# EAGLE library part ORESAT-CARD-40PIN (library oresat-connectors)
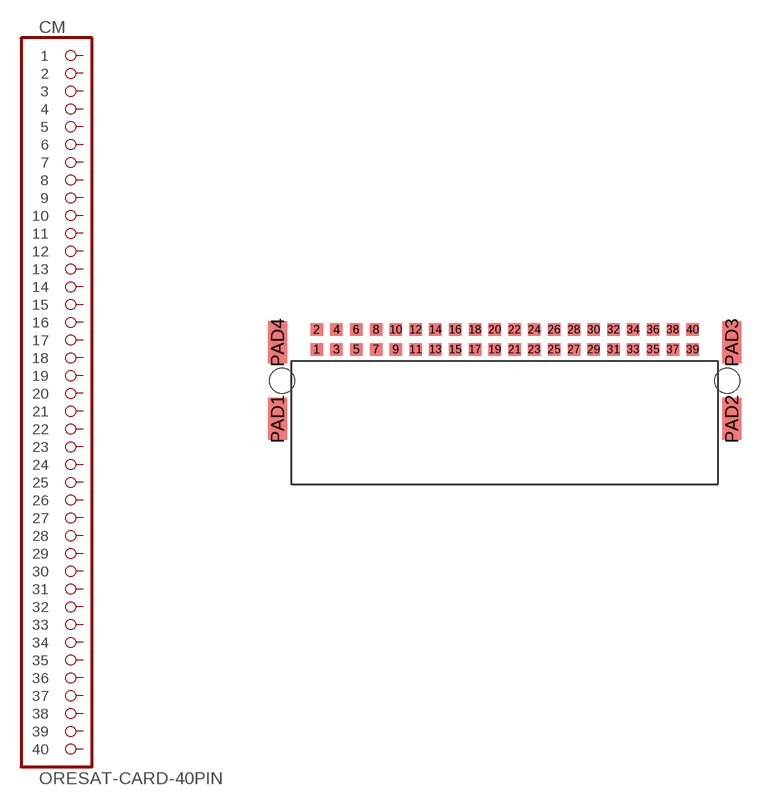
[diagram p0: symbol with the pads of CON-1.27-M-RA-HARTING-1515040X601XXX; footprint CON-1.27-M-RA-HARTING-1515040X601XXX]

Designator prefix CM

## ORESAT-CARD-40PIN  [CON-1.27-M-RA-HARTING-1515040X601XXX]
1  1  pas
2  2  pas
3  3  pas
4  4  pas
5  5  pas
6  6  pas
7  7  pas
8  8  pas
9  9  pas
10  10  pas
11  11  pas
12  12  pas
13  13  pas
14  14  pas
15  15  pas
16  16  pas
17  17  pas
18  18  pas
19  19  pas
20  20  pas
21  21  pas
22  22  pas
23  23  pas
24  24  pas
25  25  pas
26  26  pas
27  27  pas
28  28  pas
29  29  pas
30  30  pas
31  31  pas
32  32  pas
33  33  pas
34  34  pas
35  35  pas
36  36  pas
37  37  pas
38  38  pas
39  39  pas
40  40  pas

## Footprint CON-1.27-M-RA-HARTING-1515040X601XXX (pad centres in mm)
smd 0.8 x 0.8: 1 -12.065,2; 2 -12.065,3.27; 3 -10.795,2; 4 -10.795,3.27; 5 -9.525,2; 6 -9.525,3.27; 7 -8.255,2; 8 -8.255,3.27; 9 -6.985,2; 10 -6.985,3.27; 11 -5.715,2; 12 -5.715,3.27; 13 -4.445,2; 14 -4.445,3.27; 15 -3.175,2; 16 -3.175,3.27; 17 -1.905,2; 18 -1.905,3.27; 19 -0.635,2; 20 -0.635,3.27; 21 0.635,2; 22 0.635,3.27; 23 1.905,2; 24 1.905,3.27; 25 3.175,2; 26 3.175,3.27; 27 4.445,2; 28 4.445,3.27; 29 5.715,2; 30 5.715,3.27; 31 6.985,2; 32 6.985,3.27; 33 8.255,2; 34 8.255,3.27; 35 9.525,2; 36 9.525,3.27; 37 10.795,2; 38 10.795,3.27; 39 12.065,2; 40 12.065,3.27
smd 1.2 x 2.7: PAD1 -14.575,-2.45; PAD2 14.575,-2.45; PAD3 14.575,2.45; PAD4 -14.575,2.45
hole 1.6 at 14.275,0
hole 1.6 at -14.275,0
